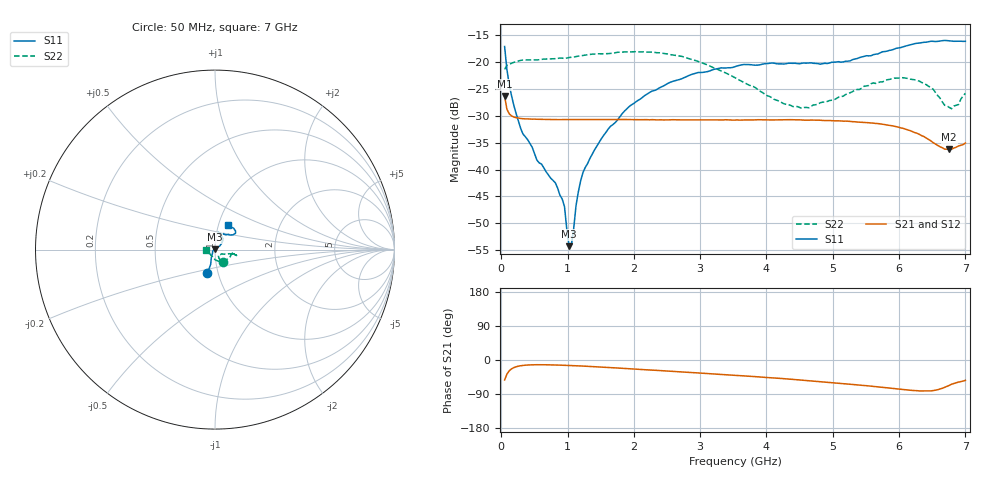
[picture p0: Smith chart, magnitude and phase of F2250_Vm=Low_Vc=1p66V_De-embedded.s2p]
! Integrated Device Technology
! Corporate Headquarters
! 6024 Silver Creek Valley Road
! San Jose, CA 95138  USA
! Phone:  1-408-284-8200
! Toll Free:  1-800-223-1366
! Webpage:  http://www.idt.com/
! Timing and RF Division
! 515 Groton Road, Suite 102
! Westford, MA 01886-6024
! Device:  F2250
! Description: Voltage Variable RF Attenuator
! Frequency:  50.0 -  6000.00 MHz
! Package:  3x3 mm Thin QFN Plastic Package: 16 pin
! Ports:  2 RF, 3 DC
!  Pin  1  = GND
!  Pin  2  = NC
!  Pin  3  = RF1  = Port 1
!  Pin  4  = NC
!  Pin  5  = GND
!  Pin  6  = GND
!  Pin  7  = GND
!  Pin  8  = GND
!  Pin  9  = NC
!  Pin 10  = RF2  = Port 2
!  Pin 11  = NC
!  Pin 12  = GND
!  Pin 13  = GND
!  Pin 14  = VCNTRL
!  Pin 15  = VDD
!  Pin 16  = VMODE
! Vcntrl:  1.660 Volts
! Vmode:  +0.000 Volts
! Vdd:  +3.30  Volts
! Current:  1.187 mA
! Data:  The device was measured on a the F2250 evaluation board which has
!  individual transmission lines to the RF pins.  Data was collected
!  using a calibrated network analyzer.  The evaluation board was
!  de-embedded using a TRL calibration technique.
!  The reference plane is the edge of the package pin.
! Misc:  SN 10
!  Action Tracker AT0258
! Date Measured:  2014-11-26
! Date:  2015-10-15  MJV
! Note:
!  Integrated Device Technology supplies this data as a sample of measured
!  data at the package pin for this product.  Your particular data for this
!  product may vary.
!  Data was taken at 25 degrees C.
!  Integrated Device Technology reserves the right to change this data at anytime.
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# GHz S dB R 50
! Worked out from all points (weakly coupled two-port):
!   201 points, 50 MHz to 7 GHz, reference 50 ohm
!   highest |S21| = -26.37 dB at 50 MHz (marker M1); lowest = -36.2 dB at 6.757 GHz (marker M2)
!   lowest |S11| = -54.2 dB at 1.023 GHz (marker M3), VSWR 1.00, Z = 49.9 + j0.141 ohm
!   |S11| at or under -10 dB: start of sweep to end of sweep
!   |S22| runs from -28.7 to -18.1 dB; largest |S21 - S12| = 0.00012
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0.05  -17.15 -107.8  -26.37 -52.7  -26.38 -52.7  -21.41 -56.5
0.1195  -24.20 -110.4  -29.64 -28.6  -29.66 -28.6  -20.41 -16.8
0.29325  -32.40 -124.9  -30.51 -15.1  -30.52 -15.1  -19.72 -9.4
0.8145  -42.45 174.2  -30.72 -13.2  -30.73 -13.1  -19.41 -11.0
0.91875  -45.47 157.1  -30.71 -13.8  -30.72 -13.7  -19.30 -12.5
0.9535  -46.89 172.5  -30.72 -13.9  -30.72 -13.9  -19.39 -12.5
1.023  -54.23 133.4  -30.71 -14.4  -30.72 -14.4  -19.19 -12.4
1.05775  -54.02 100.3  -30.71 -14.6  -30.73 -14.6  -19.16 -12.6
1.12725  -46.68 49.8  -30.72 -15.1  -30.73 -15.1  -19.01 -13.4
1.2315  -40.57 36.9  -30.71 -16.0  -30.72 -16.0  -18.82 -14.6
1.6485  -31.96 39.2  -30.74 -20.0  -30.71 -20.1  -18.43 -15.1
1.9265  -28.32 39.6  -30.72 -23.0  -30.73 -23.0  -18.15 -15.3
2.37825  -24.87 46.1  -30.77 -27.8  -30.77 -27.8  -18.31 -14.5
2.93425  -22.09 59.1  -30.79 -33.7  -30.78 -33.7  -19.77 -13.7
3.525  -20.89 71.9  -30.81 -40.4  -30.80 -40.5  -22.94 -20.9
4.25475  -20.40 77.5  -30.76 -49.1  -30.77 -49.1  -27.74 -38.7
4.7065  -20.27 72.0  -30.81 -55.5  -30.81 -55.5  -28.00 -57.0
5.85325  -17.87 40.1  -31.79 -74.2  -31.77 -74.3  -23.26 -66.7
6.305  -16.50 40.3  -33.46 -81.6  -33.45 -81.7  -23.57 -75.7
6.75675  -16.09 50.9  -36.23 -67.0  -36.25 -66.9  -28.46 -129.7
6.89575  -16.14 56.8  -35.62 -58.3  -35.63 -58.2  -27.93 -162.6
7  -16.18 63.0  -35.07 -53.8  -35.06 -53.8  -25.85 180.0
